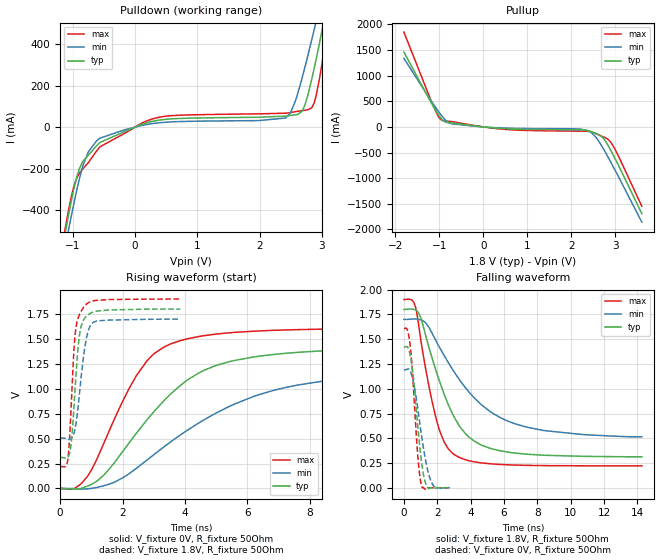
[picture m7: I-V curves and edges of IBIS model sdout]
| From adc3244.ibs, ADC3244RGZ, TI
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|   sdout Model
[Model]   sdout
Model_type   Output
Polarity   Non-Inverting
Vmeas = 0.9
Vref = 0
Cref = 2pF
Rref = 50
|   typ   min   max
|   (nom PVT)   (fast PVT)   (slow PVT)
C_comp   1.585e-12   1.577e-12   1.601e-12
| Where nom  PVT is Nominal Process, 1.8V, 27C
|   Fast PVT is Strong Process,  1.9V, -40C
|   Slow PVT is Weak Process,   1.7V, 125C
[Voltage Range]   1.8   1.7   1.9
|Junction Temperature
[Temperature Range]   27   125   -40
[Pullup Reference]   1.8   1.7   1.9
[Pulldown Reference]   0   0   0
[Power Clamp Reference]   1.8   1.7   1.9
[GND Clamp Reference]   0   0   0
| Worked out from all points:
|   slope of the pulldown table from 0 to 0.27 V, typ, clamps not added: 9.98 ohm
|   slope of the pullup table from 0 to 0.27 V, typ, clamps not added: 12.6 ohm
|   falling waveform, V_fixture 1.8V, R_fixture 50Ohm: 20-80 % time 2.03ns typ, 3.34ns min, 1.23ns max; typ from 1.8 V to 0.313 V
|   rising waveform, V_fixture 0V, R_fixture 50Ohm: 20-80 % time 2.52ns typ, 3.87ns min, 1.59ns max; typ from 0 V to 1.42 V
|   rising waveform, V_fixture 1.8V, R_fixture 50Ohm: 20-80 % time 208ps typ, 267ps min, 176ps max; typ from 0.312 V to 1.8 V
|   falling waveform, V_fixture 0V, R_fixture 50Ohm: 20-80 % time 487ps typ, 650ps min, 370ps max; typ from 1.42 V to 0 V
[Pulldown]
|   Voltage   I(typ)   I(min)   I(max)
-1.8V     -1.716A    -1.71A     -1.75A
-1.141V   -546.3mA   -614.3mA   -526.1mA
-1.072V   -434.4mA   -506.6mA   -411.6mA
-891.8mV  -201.3mA   -250.4mA   -223mA
-561.2mV  -74.02mA   -53.15mA   -95mA
375.5mV   33.19mA    20.5mA     46.78mA
2.418V    53.15mA    44.04mA    67.3mA
2.677V    75.38mA    230.8mA    79.49mA
2.837V    230.8mA    421.6mA    93.27mA
2.997V    458.5mA    625.5mA    297.9mA
3.085V    591.4mA    740.3mA    467.6mA
3.6V      1.402A     1.428A     1.556A
[Pullup]
|   Voltage   I(typ)   I(min)   I(max)
-1.8V     1.461A     1.338A     1.849A
-1.188V   483.5mA    515.7mA    523.5mA
-968.7mV  177.6mA    246.2mA    149.1mA
-848mV    91.7mA     125.1mA    114.8mA
-705.2mV  77.37mA    59.32mA    102.1mA
556mV     -37mA      -25.17mA   -52.09mA
2.205V    -56.63mA   -41.93mA   -82.72mA
2.448V    -91.97mA   -110.2mA   -95.3mA
2.705V    -201.5mA   -393.7mA   -188.8mA
2.892V    -452.7mA   -681.9mA   -295.7mA
3.085V    -777.1mA   -996.2mA   -597.5mA
3.6V      -1.695A    -1.859A    -1.549A
[Ramp]
R_load = 50
|   typ   min   max
dV/dt_r   0.851337/2.50845e-09   0.712078/3.86157e-09   0.964599/1.58274e-09
dV/dt_f   0.892879/2.02801e-09   0.716285/3.40077e-09   1.0073/1.23218e-09
[Falling Waveform]
V_fixture = 1.8V
V_fixture_min = 1.7V
V_fixture_max = 1.9V
R_fixture = 50Ohm
|   Time   V(typ)   V(min)   V(max)
0s        1.8V       1.7V       1.9V
468ps     1.805V     1.704V     1.898V
694ps     1.796V     1.704V     1.826V
994ps     1.724V     1.698V     1.515V
1.93ns    1.18V      1.482V     701mV
2.424ns   940.7mV    1.333V     460.1mV
2.988ns   722.6mV    1.177V     339mV
4.166ns   477.3mV    917.6mV    264.1mV
6.564ns   352.6mV    652.4mV    230mV
14.27ns   313mV      514.9mV    221.3mV
[Rising Waveform]
V_fixture = 0V
V_fixture_min = 0V
V_fixture_max = 0V
R_fixture = 50Ohm
|   Time   V(typ)   V(min)   V(max)
0s        1.319nV    49.54nV    304.1pV
634ps     -2.115mV   -6.126mV   37.49mV
1.198ns   78.82mV    11.61mV    310.1mV
2.128ns   422.9mV    131.1mV    953.7mV
2.778ns   686.5mV    284.1mV    1.279V
3.944ns   1.057V     556.3mV    1.491V
5.54ns    1.281V     840.3mV    1.564V
8.336ns   1.379V     1.072V     1.597V
11.64ns   1.408V     1.149V     1.606V
20ns      1.419V     1.187V     1.608V
[Rising Waveform]
V_fixture = 1.8V
V_fixture_min = 1.7V
V_fixture_max = 1.9V
R_fixture = 50Ohm
|   Time   V(typ)   V(min)   V(max)
0s        311.8mV    504.5mV    221.2mV
228ps     307.7mV    494.4mV    258mV
326ps     388.8mV    494.2mV    648.4mV
418ps     702.8mV    532.2mV    1.255V
486ps     1.036V     612.1mV    1.563V
612ps     1.521V     931.9mV    1.74V
746ps     1.689V     1.317V     1.814V
890ps     1.741V     1.573V     1.861V
1.056ns   1.769V     1.666V     1.882V
3.848ns   1.799V     1.698V     1.9V
[Falling Waveform]
V_fixture = 0V
V_fixture_min = 0V
V_fixture_max = 0V
R_fixture = 50Ohm
|   Time   V(typ)   V(min)   V(max)
0s        1.42V      1.191V     1.608V
192ps     1.426V     1.196V     1.601V
396ps     1.322V     1.174V     1.41V
584ps     1.09V      1.057V     983.7mV
832ps     625.9mV    801.4mV    324.6mV
978ps     375.8mV    623mV      87.61mV
1.054ns   267.3mV    533.1mV    23.52mV
1.342ns   30.03mV    243mV      -13.28mV
1.746ns   -5.389mV   27.05mV    1.056mV
2.742ns   422.5uV    1.407mV    135.8uV
